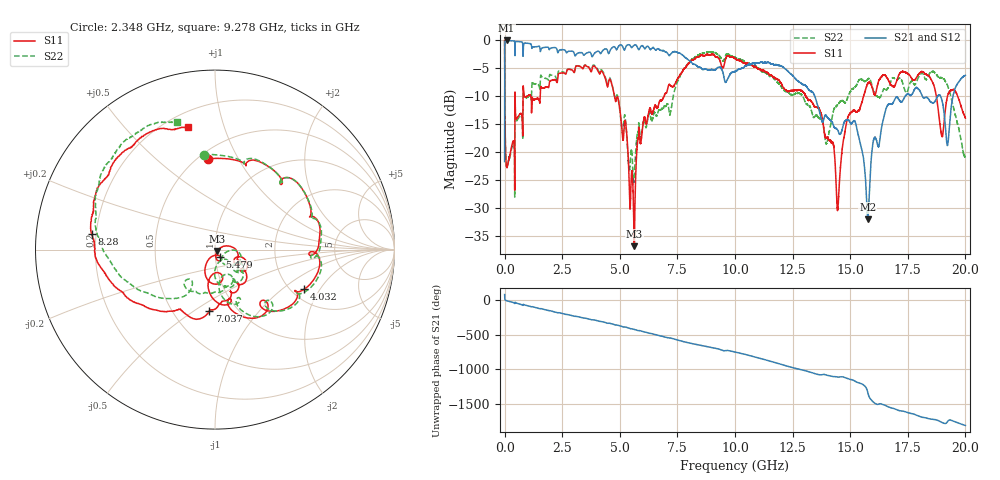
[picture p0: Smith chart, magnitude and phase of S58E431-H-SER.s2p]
!{S58E431}
!Johanson Technology Inc.
!www.johansontechnology.com
!Test Board Conditions:
!Substrate Type  RO4350B
!Substrate Thickness  60 mil
!Substrate Dk  3.66
!TL Type: GCPW
!TL Trace Width  115 mil
!TL Gap  52 mil
!Electrode orientation  Horizontal
!DUT TOPOLOGY	SERIES
!Mounting Pad LxW  55x428 mil
! Created Wed Apr 14 11:49:14 2021
# mhz S ma R 50
! 2 Port Network Data from SP1.SP block
! freq  magS11  angS11  magS21  angS21  magS12  angS12  magS22  angS22
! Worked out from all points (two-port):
!   20001 points, 300 kHz to 20 GHz, reference 50 ohm
!   highest |S21| = -0.03 dB at 84.3 MHz (marker M1); lowest = -31.9 dB at 15.77 GHz (marker M2)
!   |S21| within 3 dB of the highest: 3.692 MHz to 7.816 GHz (7.812 GHz wide, 200 % of centre)
!   lowest |S11| = -36.8 dB at 5.627 GHz (marker M3), VSWR 1.03, Z = 51.2 - j0.814 ohm
!   |S11| at or under -10 dB: 4.768 GHz to 6.923 GHz (2.154 GHz wide, 36.9 % of centre); 13.08 GHz to 15.58 GHz (2.502 GHz wide, 17.5 % of centre); 18.74 GHz to 19.22 GHz (482.5 MHz wide, 2.54 % of centre)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
!   |S22| runs from -28.0 to 0.0 dB; largest |S21 - S12| = 0.012
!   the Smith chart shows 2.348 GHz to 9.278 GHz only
!   S11 on the Smith chart (normalised r, x): 2.348 GHz: 0.56, +0.75; 4.032 GHz: 2.33, -1.46; 5.479 GHz: 1.06, -0.08; 7.037 GHz: 0.75, -0.58; 8.28 GHz: 0.18, +0.06; 9.278 GHz: 0.29, +0.76
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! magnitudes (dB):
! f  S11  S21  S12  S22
! 300 kHz  0.0  -21.7  -21.7  0.0
! 84.3 MHz  -22.6  0.0  0.0  -22.5
! 2.348 GHz  -5.9  -1.9  -1.9  -5.5
! 3.334 GHz  -4.8  -2.2  -2.2  -4.8
! 4.032 GHz  -5.3  -2.0  -2.0  -5.1
! 4.939 GHz  -10.6  -1.1  -1.1  -10.7
! 5.479 GHz  -26.4  -1.1  -1.1  -20.2
! 5.627 GHz  -36.8  -0.9  -0.9  -24.2
! 5.818 GHz  -17.4  -1.7  -1.7  -16.9
! 6.667 GHz  -11.7  -1.5  -1.5  -12.7
! 7.037 GHz  -9.3  -2.2  -2.1  -11.5
! 8.28 GHz  -3.2  -4.3  -4.3  -3.0
! 9.278 GHz  -3.1  -4.8  -4.9  -2.6
! 10 GHz  -3.2  -5.6  -5.6  -3.1
! 13.33 GHz  -11.0  -9.2  -9.1  -12.9
! 14.47 GHz  -29.9  -16.1  -15.9  -11.4
! 15.22 GHz  -12.6  -14.6  -14.6  -8.3
! 15.77 GHz  -7.7  -31.9  -32.3  -6.9
! 16.67 GHz  -7.2  -11.4  -11.5  -8.3
! 18.39 GHz  -6.3  -10.4  -10.4  -6.4
! 19.04 GHz  -16.0  -12.0  -12.0  -6.9
! 20 GHz  -13.9  -6.3  -6.2  -20.7
